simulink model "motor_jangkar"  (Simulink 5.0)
settings: Solver=ode4  StartTime=0.0  StopTime=0.5  FixedStep=0.001  RelTol=1e-6

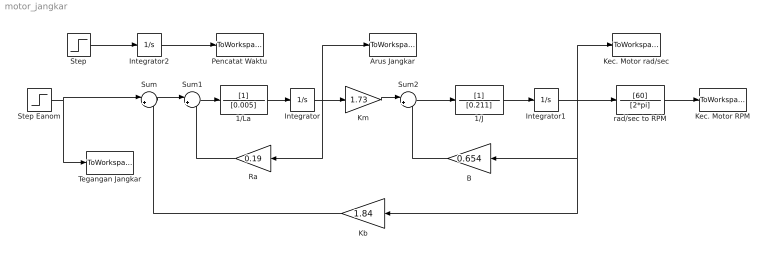
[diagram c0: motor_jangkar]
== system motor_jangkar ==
  1/J : TransferFcn  Denominator=[0.211]
  1/La : TransferFcn  Denominator=[0.005]
  Arus Jangkar : ToWorkspace  VariableName=arus  SampleTime=-1  SaveFormat=Array
  B : Gain  Orientation=left  Gain=0.654
  Integrator : Integrator
  Integrator1 : Integrator
  Integrator2 : Integrator
  Kb : Gain  Orientation=left  Gain=1.84
  Kec. Motor RPM : ToWorkspace  VariableName=rpm  SampleTime=-1  SaveFormat=Array
  Kec. Motor rad/sec : ToWorkspace  VariableName=omega  SampleTime=-1  SaveFormat=Array
  Km : Gain  Gain=1.73
  Pencatat Waktu : ToWorkspace  VariableName=time  SampleTime=-1  SaveFormat=Array
  Ra : Gain  Orientation=left  Gain=0.19
  Step : Step  Time=0  SampleTime=0
  Step Eanom : Step  Time=0.01  After=500  SampleTime=0
  Sum : Sum  Inputs=|+-
  Sum1 : Sum  Inputs=|+-
  Sum2 : Sum  Inputs=|+-
  Tegangan Jangkar : ToWorkspace  VariableName=tegangan  SampleTime=-1  SaveFormat=Array
  rad/sec to RPM : TransferFcn  Numerator=[60]  Denominator=[2*pi]
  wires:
  Step/1 -> Integrator2/1
  Integrator2/1 -> Pencatat Waktu/1
  Step Eanom/1 -> Sum/1, Tegangan Jangkar/1
  Sum/1 -> Sum1/1
  Sum1/1 -> 1/La/1
  1/La/1 -> Integrator/1
  Integrator/1 -> Km/1, Ra/1, Arus Jangkar/1
  Km/1 -> Sum2/1
  Sum2/1 -> 1/J/1
  1/J/1 -> Integrator1/1
  Integrator1/1 -> rad/sec to RPM/1, B/1, Kb/1, Kec. Motor rad/sec/1
  B/1 -> Sum2/2
  Ra/1 -> Sum1/2
  Kb/1 -> Sum/2
  rad/sec to RPM/1 -> Kec. Motor RPM/1
